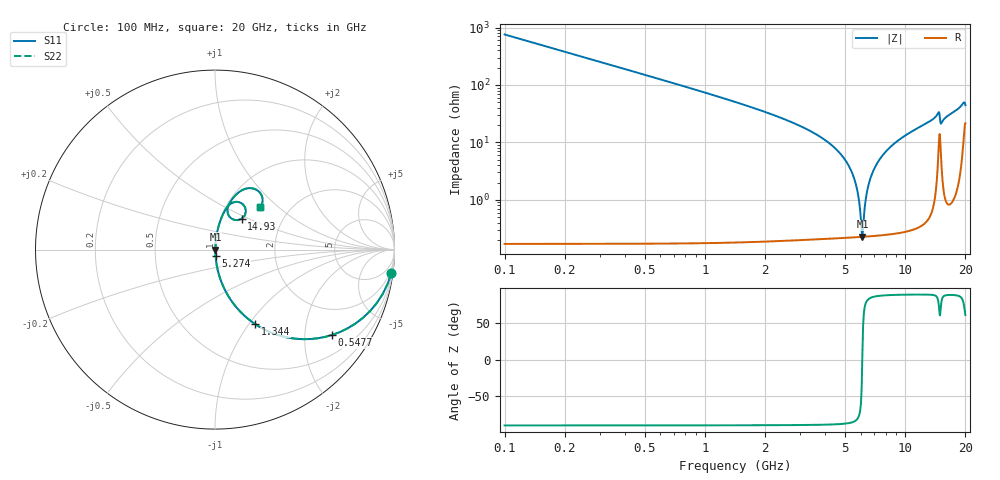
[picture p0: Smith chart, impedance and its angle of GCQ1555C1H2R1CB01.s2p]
!Murata Part Number: GCQ1555C1H2R1CB01
!These Parameters are Measured in Series Mode Connection
!Data Generated on Jan 08, 2026
!  o--ll--o
!Port1  Port2
!  o------o
!Operation Temp=25[degC], DC Bias Voltage=0[V]
!Freq. Start=100[MHz] Stop=20[GHz] 401[Steps]
# Hz S RI R 50
!Freq.(Hz) S11(Real) S11(Imag) S21(Real) S21(Imag) S12(Real) S12(Imag) S22(Real) S22(Imag)
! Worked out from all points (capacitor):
!   401 points, 100 MHz to 20 GHz, reference 50 ohm
!   read as one part in series: C = 2.1 pF near 199.5 MHz
!   lowest |Z| = 229 mohm at 6.12 GHz (marker M1)
!   series resonance near 6.112 GHz, so ESL is about 320 pH
!   S11 on the Smith chart (normalised r, x): 100 MHz: 1, -15; 547.8 MHz: 1.00, -2.75; 1.344 GHz: 1.00, -1.07; 5.274 GHz: 1.00, -0.07; 14.93 GHz: 1.26, +0.46; 20 GHz: 1.43, +0.77
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1e8  0.9829 -0.1297  0.0171 0.1297  0.0171 0.1297  0.9829 -0.1297
2.99e8  0.8646 -0.3418  0.1354 0.3418  0.1354 0.3418  0.8646 -0.3418
5.4775e8  0.6531 -0.4754  0.3469 0.4754  0.3469 0.4754  0.6531 -0.4754
1.34375e9  0.2245 -0.4156  0.7755 0.4156  0.7755 0.4156  0.2245 -0.4156
3.43325e9  0.0243 -0.1474  0.9757 0.1474  0.9757 0.1474  0.0243 -0.1474
4.5775e9  0.00739 -0.0723  0.9926 0.0723  0.9926 0.0723  0.00739 -0.0723
5.274e9  0.00354 -0.0367  0.9965 0.0367  0.9965 0.0367  0.00354 -0.0367
5.72175e9  0.00249 -0.0164  0.9975 0.0164  0.9975 0.0164  0.00249 -0.0164
5.871e9  0.00234 -0.01  0.9977 0.01  0.9977 0.01  0.00234 -0.01
6.02025e9  0.00226 -0.00375  0.9977 0.00375  0.9977 0.00375  0.00226 -0.00375
6.11975e9  0.00226 0.000331  0.9977 -0.000331  0.9977 -0.000331  0.00226 0.000331
6.41825e9  0.00243 0.0122  0.9976 -0.0122  0.9976 -0.0122  0.00243 0.0122
6.7665e9  0.00296 0.0254  0.997 -0.0254  0.997 -0.0254  0.00296 0.0254
7.91075e9  0.00671 0.0652  0.9933 -0.0652  0.9933 -0.0652  0.00671 0.0652
1.005e10  0.0199 0.1296  0.9801 -0.1296  0.9801 -0.1296  0.0199 0.1296
1.338325e10  0.0577 0.2222  0.9423 -0.2222  0.9423 -0.2222  0.0577 0.2222
1.467675e10  0.1439 0.2605  0.8561 -0.2605  0.8561 -0.2605  0.1439 0.2605
1.49255e10  0.1493 0.172  0.8507 -0.172  0.8507 -0.172  0.1493 0.172
1.51245e10  0.0851 0.1787  0.9149 -0.1787  0.9149 -0.1787  0.0851 0.1787
1.67165e10  0.092 0.2758  0.908 -0.2758  0.908 -0.2758  0.092 0.2758
1.925375e10  0.1982 0.3425  0.8018 -0.3425  0.8018 -0.3425  0.1982 0.3425
2e10  0.2531 0.238  0.7469 -0.238  0.7469 -0.238  0.2531 0.238
